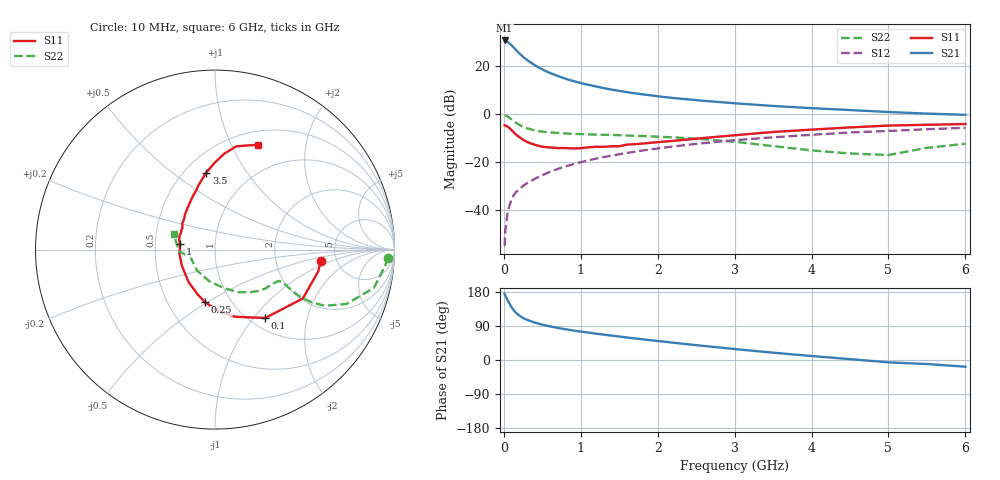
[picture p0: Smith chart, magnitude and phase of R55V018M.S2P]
! SIEMENS Small Signal Semiconductors
! BFR183
! Si NPN RF Bipolar Junction Transistor in SOT23
! VCE = 5 V  IC = 18 mA
! Common Emitter S-Parameters:  May  1996
# GHz  S  MA  R  50
!  f  S11  S21  S12  S22
! GHz  MAG  ANG  MAG  ANG  MAG  ANG  MAG  ANG
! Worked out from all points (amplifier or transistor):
!   36 points, 10 MHz to 6 GHz, reference 50 ohm
!   highest |S21| = 30.8 dB at 10 MHz (marker M1)
!   |S21| within 3 dB of that: start of sweep to 128.8 MHz
!   unconditionally stable (mu >= 1): 633.8 MHz to 2.444 GHz
!   at 250 MHz: K = 0.77, MSG = 26.9 dB, |S12| = -29.8 dB
!   at 1.4 GHz: K = 1.04, MAG = 12.5 dB, |S12| = -17.2 dB
!   at 6 GHz: K = 0.90, MSG = 2.7 dB, |S12| = -5.6 dB
!   S11 on the Smith chart (normalised r, x): 10 MHz: 3.77, -0.74; 100 MHz: 1.17, -1.15; 250 MHz: 0.76, -0.49; 1 GHz: 0.67, +0.04; 3.5 GHz: 0.63, +0.67; 6 GHz: 0.65, +1.27
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0.01  0.5941 -6.1  34.87 174.9  0.0018 86.6  0.966 -2.7
0.02  0.5873 -12.1  34.73 170.0  0.0038 86.2  0.9513 -5.6
0.05  0.5601 -29.1  32.87 157.0  0.0094 76.9  0.9102 -13.6
0.1  0.4728 -53.7  27.66 139.4  0.0173 71.7  0.7921 -22.5
0.15  0.3911 -73.1  22.7 126.0  0.0234 67.9  0.6865 -27.1
0.2  0.3397 -87.7  18.85 117.5  0.0276 67.6  0.6091 -28.7
0.25  0.2982 -100.7  15.87 110.9  0.0325 67.2  0.5538 -29.0
0.3  0.2673 -111.4  13.68 105.9  0.0368 68.2  0.5164 -28.7
0.4  0.2331 -129.1  10.68 99.0  0.0454 69.5  0.4672 -27.5
0.5  0.2126 -142.5  8.659 93.2  0.0543 70.0  0.4384 -26.5
0.6  0.2053 -154.1  7.318 88.8  0.0639 70.4  0.4228 -26.0
0.7  0.1994 -164.5  6.347 84.7  0.0731 70.6  0.4114 -26.0
0.8  0.1996 -173.8  5.572 81.2  0.0826 70.3  0.4018 -26.1
1  0.1981 171.4  4.523 75.1  0.1011 69.6  0.3902 -27.0
1.1  0.207 164.9  4.148 72.3  0.1109 69.0  0.3856 -28.2
1.3  0.2114 154.1  3.536 66.9  0.1298 67.2  0.3767 -30.0
1.6  0.2354 140.7  2.917 59.3  0.158 64.6  0.3635 -34.0
2.2  0.2817 122.2  2.203 45.7  0.2151 58.6  0.3334 -43.7
3.5  0.4318 96.5  1.504 19.3  0.3341 42.7  0.219 -77.3
4.5  0.5369 84.5  1.236 2.3  0.4212 30.3  0.1537 -130.6
5.5  0.6097 72.2  1.043 -10.6  0.4931 18.6  0.2014 -177.2
6  0.6318 67.6  0.983 -17.7  0.5271 11.1  0.245 159.4
